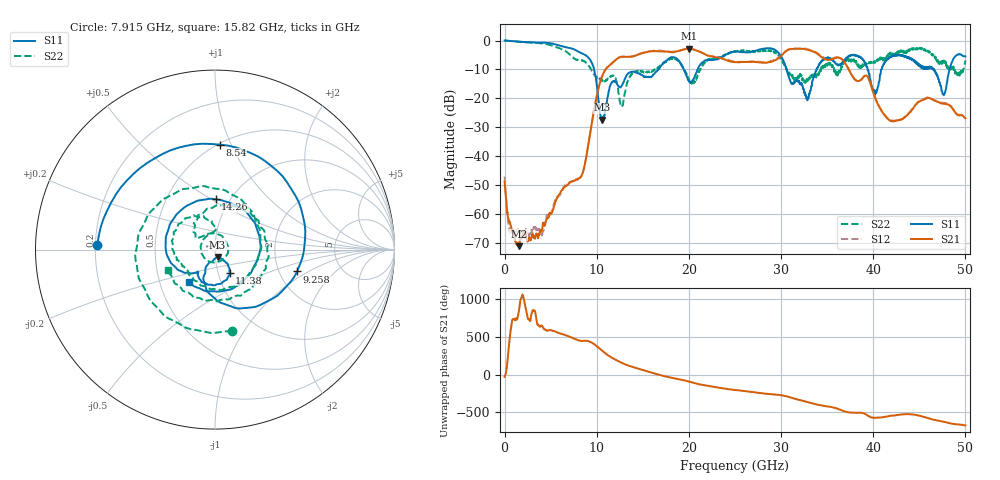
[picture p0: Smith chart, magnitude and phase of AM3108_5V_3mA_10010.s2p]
# Hz S DB R 50.0
!freq dBS11 angS11 dBS21 angS21 dBS12 angS12 dBS22 angS22
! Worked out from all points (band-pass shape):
!   1601 points, 10 MHz to 50 GHz, reference 50 ohm
!   highest |S21| = -2.75 dB at 20.04 GHz (marker M1); lowest = -71.1 dB at 1.541 GHz (marker M2)
!   |S21| within 3 dB of the highest: 12.52 GHz to 22.92 GHz (10.4 GHz wide, 58.7 % of centre); 29.86 GHz to 34.42 GHz (4.565 GHz wide, 14.2 % of centre)
!   lowest |S11| = -27.4 dB at 10.6 GHz (marker M3), VSWR 1.09, Z = 51.3 - j4.15 ohm
!   |S11| at or under -10 dB: 9.715 GHz to 16.69 GHz (6.979 GHz wide, 52.9 % of centre); 30.61 GHz to 33.84 GHz (3.233 GHz wide, 10 % of centre); 46.62 GHz to 48.29 GHz (1.666 GHz wide, 3.51 % of centre)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
!   |S22| runs from -23.0 to 0.0 dB; largest |S21 - S12| = 0.026
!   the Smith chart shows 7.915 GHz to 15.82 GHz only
!   S11 on the Smith chart (normalised r, x): 7.915 GHz: 0.21, +0.02; 8.54 GHz: 0.51, +0.91; 9.258 GHz: 2.51, -0.79; 11.38 GHz: 1.14, -0.30; 14.26 GHz: 0.86, +0.52; 15.82 GHz: 0.70, -0.27
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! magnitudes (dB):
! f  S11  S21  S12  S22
! 10 MHz  0.0  -48.8  -47.0  0.0
! 603.6 MHz  -0.1  -62.9  -65.8  -0.2
! 1.541 GHz  -0.3  -71.1  -65.8  -0.5
! 4.072 GHz  -0.7  -65.6  -67.3  -1.0
! 7.915 GHz  -3.7  -47.9  -48.1  -6.7
! 8.352 GHz  -4.3  -46.8  -46.6  -6.8
! 8.54 GHz  -4.7  -45.2  -45.1  -7.0
! 9.258 GHz  -6.5  -32.7  -32.7  -9.4
! 10.6 GHz  -27.4  -12.3  -12.3  -13.7
! 11.38 GHz  -16.4  -8.6  -8.5  -12.9
! 12.73 GHz  -15.6  -5.6  -5.5  -23.0
! 14.26 GHz  -11.0  -5.2  -4.9  -10.6
! 15.82 GHz  -12.7  -3.7  -3.6  -10.8
! 16.69 GHz  -10.0  -3.7  -3.4  -9.4
! 20.04 GHz  -14.2  -2.8  -2.6  -13.7
! 25 GHz  -3.7  -7.4  -7.3  -3.8
! 33.35 GHz  -15.5  -3.6  -3.4  -12.7
! 37.88 GHz  -4.9  -13.0  -12.9  -6.5
! 40.22 GHz  -18.6  -20.0  -19.8  -7.6
! 41.69 GHz  -6.1  -27.4  -27.1  -5.3
! 47.66 GHz  -18.9  -21.9  -21.6  -7.7
! 50 GHz  -5.5  -26.9  -26.4  -6.9
